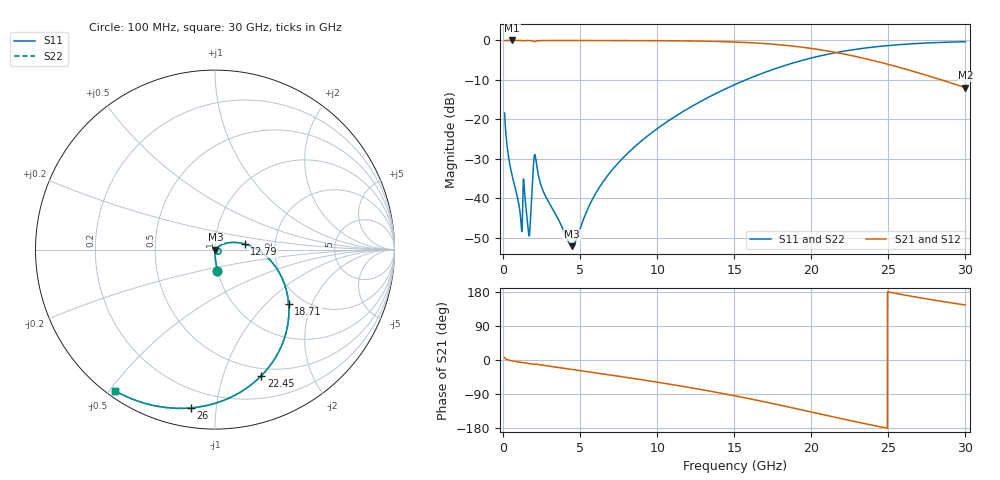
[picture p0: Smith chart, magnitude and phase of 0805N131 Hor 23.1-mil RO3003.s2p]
# GHz S MA R 50
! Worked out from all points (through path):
!   3201 points, 100 MHz to 30 GHz, reference 50 ohm
!   highest |S21| = -0.01 dB at 595.2 MHz (marker M1); lowest = -12.0 dB at 30 GHz (marker M2)
!   group delay of S21, straight-line fit = 20.9 ps
!   lowest |S11| = -52.1 dB at 4.473 GHz (marker M3), VSWR 1.00, Z = 50.2 - j0.109 ohm
!   |S11| at or under -10 dB: start of sweep to 15.74 GHz
!   |S22| runs from -52.1 to -0.3 dB; largest |S21 - S12| = 0
!   S11 on the Smith chart (normalised r, x): 100 MHz: 1.00, -0.24; 12.79 GHz: 1.39, +0.09; 18.71 GHz: 1.68, -1.38; 22.45 GHz: 0.42, -1.34; 26 GHz: 0.10, -0.85; 30 GHz: 0.02, -0.52
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0.1  0.1204 -83.5  0.9924 6.4  0.9924 6.4  0.1204 -83.5
0.3522812  0.03381 -89.1  0.9988 -0.0  0.9988 -0.0  0.03381 -89.1
0.5952188  0.01917 -90.0  0.999 -2.3  0.999 -2.3  0.01917 -90.0
1.118469  0.006182 -81.7  0.9984 -5.9  0.9984 -5.9  0.006182 -81.7
1.426813  0.01006 -76.6  0.9963 -7.5  0.9963 -7.5  0.01006 -76.6
1.660406  0.003496 -42.6  0.997 -9.2  0.997 -9.2  0.003496 -42.6
1.772531  0.005069 15.4  0.9954 -10.1  0.9954 -10.1  0.005069 15.4
1.987437  0.02894 3.7  0.972 -11.6  0.972 -11.6  0.02894 3.7
2.11825  0.03182 -54.3  0.9767 -10.6  0.9767 -10.6  0.03182 -54.3
2.650844  0.01174 -87.7  0.9965 -14.2  0.9965 -14.2  0.01174 -87.7
4.472875  0.002476 -26.1  0.9974 -24.9  0.9974 -24.9  0.002476 -26.1
5.089563  0.004636 27.7  0.9972 -28.5  0.9972 -28.5  0.004636 27.7
6.911594  0.02086 42.5  0.9966 -39.3  0.9966 -39.3  0.02086 42.5
10.06978  0.07794 28.2  0.9927 -58.9  0.9927 -58.9  0.07794 28.2
12.78881  0.1674 10.8  0.9805 -77.5  0.9805 -77.5  0.1674 10.8
15.05  0.2765 -5.8  0.9546 -94.6  0.9546 -94.6  0.2765 -5.8
18.71275  0.5107 -36.5  0.8514 -125.7  0.8514 -125.7  0.5107 -36.5
20.03956  0.6013 -48.4  0.79 -137.6  0.79 -137.6  0.6013 -48.4
22.45025  0.7487 -69.9  0.6528 -159.2  0.6528 -159.2  0.7487 -69.9
25.01978  0.8621 -91.2  0.4958 179.4  0.4958 179.4  0.8621 -91.2
26.00088  0.8927 -98.8  0.4393 171.9  0.4393 171.9  0.8927 -98.8
30  0.9641 -125.5  0.2523 145.1  0.2523 145.1  0.9641 -125.5
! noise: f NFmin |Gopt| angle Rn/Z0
0.1  0.0004171  0.8561  0.6468  0.0006192
3.417  0.006943  0.7273  19.13  0.004926
6.743  0.01062  0.6676  37.1  0.00554
10.06  0.01477  0.6562  54  0.006577
13.39  0.01949  0.6634  69.75  0.007613
16.7  0.02522  0.6829  84.32  0.008712
20.03  0.03264  0.712  98  0.009976
23.35  0.0428  0.7491  111  0.01151
26.67  0.05769  0.7929  123.7  0.01341
30  0.08109  0.8405  136.3  0.01562
